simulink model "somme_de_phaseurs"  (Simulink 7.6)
settings: Solver=ode23tb  StartTime=0.0  StopTime=0.006  RelTol=1e-3
InitFcn:
  | clc, close all
StopFcn:
  | close all
  | load somme_2_sinusoïdes.mat
  | plot(x(1,:),x(2,:),x(1,:),x(3,:),x(1,:),x(4,:))
  | grid
  | title('Somme instantanée de 2 sinusoïdes')
  | xlabel('temps')
libraries: powerlib x8

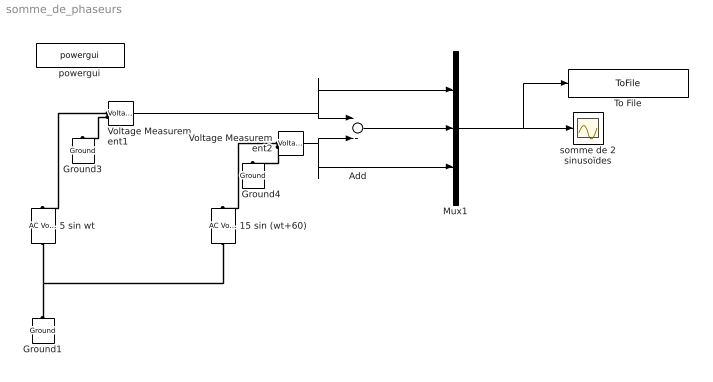
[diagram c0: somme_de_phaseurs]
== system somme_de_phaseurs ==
  15 sin (wt+60) : powerlib/Electrical Sources/AC Voltage Source  DialogController=POWERSYS.PowerSysDialog  SystemSampleTime=-1  Amplitude=15  Phase=60  Frequency=60  SampleTime=0  Measurements=None
  5 sin wt : powerlib/Electrical Sources/AC Voltage Source  DialogController=POWERSYS.PowerSysDialog  SystemSampleTime=-1  Amplitude=5  Phase=0  Frequency=60  SampleTime=0  Measurements=None
  Add : Sum
  Ground1 : powerlib/Elements/Ground  DialogController=POWERSYS.PowerSysDialog  PhysicalDomain=powersysdomain  SubClassName=unknown  LeftPortType=p1  RightPortType=p1  LConnTagsString=a
  Ground3 : powerlib/Elements/Ground  DialogController=POWERSYS.PowerSysDialog  PhysicalDomain=powersysdomain  SubClassName=unknown  LeftPortType=p1  RightPortType=p1  LConnTagsString=a
  Ground4 : powerlib/Elements/Ground  DialogController=POWERSYS.PowerSysDialog  PhysicalDomain=powersysdomain  SubClassName=unknown  LeftPortType=p1  RightPortType=p1  LConnTagsString=a
  Mux1 : Mux  Inputs=3
  To File : ToFile  Filename=somme_2_sinusoïdes  MatrixName=x
  Voltage Measurement1 : powerlib/Measurements/Voltage Measurement  DialogController=POWERSYS.PowerSysDialog  SystemSampleTime=-1  PhasorSimulation=off  OutputType=Complex  PSBequivalent=0
  Voltage Measurement2 : powerlib/Measurements/Voltage Measurement  DialogController=POWERSYS.PowerSysDialog  SystemSampleTime=-1  PhasorSimulation=off  OutputType=Complex  PSBequivalent=0
  powergui : powerlib/powergui  SystemSampleTime=-1  SimulationMode=Continuous  SampleTime=0  frequency=60  SPID=off  DisableSnubberDevices=off  DisableRonSwitches=off  DisableVfSwitches=off  SwTol=0  Interpol=off  frequencyindice=60  echomessages=off  HookPort=off  DisplayEquations=off  FunctionMessages=off  EnableUseOfTLC=off  x0status=blocks  RestoreLinks=warning  ResistiveCurrentMeasurement=off  Frange=[0:2:500]  Ylog=off  Xlog=on  ShowGrid=off  save=off  variable=ZData  ZoomFFT=on  StartTime=0.0  cycles=1  DisplayStyle=1  fundamental=60  FreqAxis=off  MaxFrequency=1000  frequencyindicesteady=1  RmsSteady=1  display=off  Ts=0  methode=off
  somme de 2 sinusoïdes : Scope
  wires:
  Voltage Measurement2/1 -> Add/2, Mux1/3
  Voltage Measurement1/1 -> Add/1, Mux1/1
  Add/1 -> Mux1/2
  Mux1/1 -> somme de 2 sinusoïdes/1, To File/1
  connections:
  Voltage Measurement1/LConn1 -- 5 sin wt/RConn1
  Voltage Measurement1/LConn2 -- Ground3/LConn1
  Voltage Measurement2/LConn1 -- 15 sin (wt+60)/RConn1
  5 sin wt/LConn1 -- Ground1/LConn1 -- 15 sin (wt+60)/LConn1
  Voltage Measurement2/LConn2 -- Ground4/LConn1
